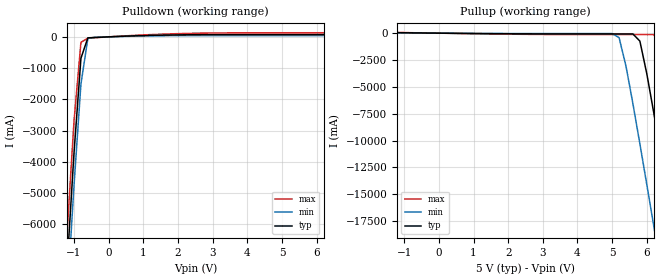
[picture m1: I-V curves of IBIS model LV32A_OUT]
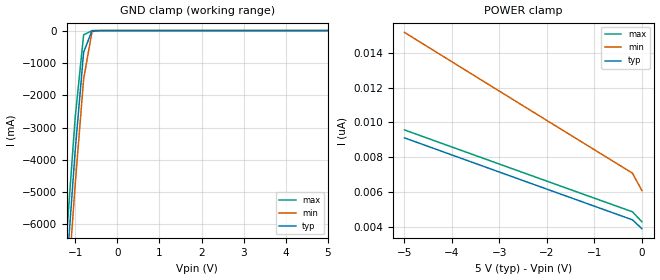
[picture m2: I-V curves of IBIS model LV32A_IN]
|   TEXAS INSTRUMENTS INCORPORATED
|   Advanced Bus Interface Group
|   IBIS Model of LV32A (Vcc=5V)
|   CMOS Quadruple 2-Input Positive-OR Gate
|   SOIC 14-pin (D) Package
[IBIS Ver]   1.1
[File Name]   lv32a_5.ibs
[File Rev]   2.0
[Date]   9/6/97
[Source]   File originated at Texas Instruments, Inc.
[Notes]   The following is an IBIS list for the LV32A.
|   - All test data contained in this file are derived from
|   hspice(tm) simulations.
|   - File created by Teruo Ishii, SLL Applications.
[Disclaimer] Property of Texas Instruments Incorporated.  Unauthorized
   reproduction and/or distribution is strictly prohibited.
   This product is protected under copyright law.
   Created 1997, (C) Copyright 1997, Texas Instruments Inc.,
   All Rights Reserved
   UNLESS THERE IS A SIGNED, WRITTEN AGREEMENT TO THE
   CONTRARY, TEXAS INSTRUMENTS ("TI") IS PROVIDING THE IBIS
   MODELS "AS IS" AND WITHOUT ANY WARRANTY, EXPRESSED OR
   IMPLIED.  TI assumes no liability for:
   1) the accuracy of the IBIS models provided to your
   company;
   2) the proper functioning of these IBIS models in your
   design or for any resulting applications; or
   3) infringement of patents, copyrights or intellectual
   property rights resulting from your use of these IBIS
   models.
   TI provides IBIS Models as a service to our customers.
   You and your company shall not distribute, sell or give
   these models to anyone else without prior written
   permission from TI.
   TI reserves the right to make changes to our products or
   to discontinue any semiconductor product or service
   without notice, and advises our customers to obtain the
   latest version of relevant information to verify, before
   placing orders, that the information being relied on is
   current.
   Please be aware that your receipt and use of the IBIS
   information provided shall serve as acceptance of these
   terms and conditions.  If you do not accept these terms,
   you should return or destroy the IBIS models and any
   other accompanying information immediately.
[Component]   LV32A(Positive-OR Gate)
[Manufacturer]  Texas Instruments
[Package]
|   typ   min   max
R_pkg   0.020   0.018   0.021
L_pkg   3.17nH   2.22nH   4.32nH
C_pkg   0.35pF   0.20pF   0.50pF
[Pin]   signal_name   model_name   R_pin   L_pin   C_pin
1   1A   LV32A_IN   0.018   4.30nH   0.50pF
2   1B   LV32A_IN   0.021   3.39nH   0.43pF
3   1Y   LV32A_OUT   0.019   2.24nH   0.26pF
4   2A   LV32A_IN   0.020   2.27nH   0.21pF
5   2B   LV32A_IN   0.020   2.22nH   0.20pF
6   2Y   LV32A_OUT   0.021   3.43nH   0.38pF
7   GND   GND   0.020   4.32nH   0.50pF
8   3Y   LV32A_OUT   0.020   4.32nH   0.50pF
9   3A   LV32A_IN   0.021   3.43nH   0.38pF
10   3B   LV32A_IN   0.020   2.22nH   0.20pF
11   4Y   LV32A_OUT   0.020   2.27nH   0.21pF
12   4A   LV32A_IN   0.019   2.24nH   0.26pF
13   4B   LV32A_IN   0.021   3.39nH   0.43pF
14   VCC   POWER   0.018   4.30nH   0.50pF
| Models and submodels in the file (2): LV32A_OUT (Output), LV32A_IN (Input)
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|   Model LV32A_OUT
[Model]   LV32A_OUT
Model_type   Output
Polarity   Non-Inverting
|variable   typ   min   max
C_comp   4.0pF   NA   NA
[Voltage range]   5.0   4.5   5.5
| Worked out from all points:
|   slope of the pulldown table from 0 to 0.75 V, typ, clamps not added: 23.2 ohm
|   slope of the pullup table from 0 to 0.75 V, typ, clamps not added: 29.8 ohm
[Pulldown]
|   Voltage   I(typ)   I(min)   I(max)
-5V       -81.99A    -82.92A    -81.08A
-1.2V     -7.334A    -8.394A    -6.29A
-1V       -3.716A    -4.76A     -2.696A
-800mV    -684.6mA   -1.507A    -174.2mA
-600mV    -32.04mA   -49.56mA   -44.95mA
-400mV    -20.26mA   -14.47mA   -29.3mA
400mV     18.84mA    13.27mA    27.19mA
2.4V      67.49mA    39.34mA    113mA
6.8V      78.69mA    44.99mA    135.4mA
10V       118mA      69.49mA    191.8mA
[Pullup]   | Note: Vtable = Vcc - Voutput
|   Voltage   I(typ)   I(min)   I(max)
-5V       63.18mA    37.18mA    178.6mA
5V        -72.29mA   -39.76mA   -130.3mA
5.2V      -72.34mA   -419.6mA   -130.3mA
5.4V      -72.63mA   -3.083A    -130.4mA
5.6V      -75.88mA   -6.59A     -130.4mA
5.8V      -740.7mA   -10.3A     -130.8mA
6.2V      -7.404A    -17.94A    -139.2mA
6.4V      -11.17A    -21.82A    -1.238A
6.8V      -18.88A    -29.62A    -8.294A
7.2V      -26.69A    -37.47A    -15.98A
7.4V      -30.61A    -41.4A     -19.88A
10V       -82.06A    -92.89A    -71.28A
[Ramp]
|Variable   typ   min   max
dV/dt_r   1.7468E+00/1.4220E-09  1.1029E+00/2.3636E-09  2.3227E+00/7.4065E-10
dV/dt_f   1.8621E+00/1.6013E-09  1.1972E+00/2.4256E-09  2.4573E+00/1.0037E-09
|   Model LV32A_IN
[Model]   LV32A_IN
Model_type   Input
Polarity   Non-Inverting
Vinl = 1.5V
Vinh = 3.5V
|variable   typ   min   max
C_comp   3.3pF   NA   NA
[Voltage Range]   5.0   4.5   5.5
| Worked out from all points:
|   GND clamp passes 1 mA (typ) near -0.46 V on its own axis
[GND_Clamp]
|   Voltage   I(typ)   I(min)   I(max)
-5V       -82A       -82.93A    -81.1A
-1.2V     -7.333A    -8.394A    -6.288A
-1V       -3.712A    -4.759A    -2.688A
-800mV    -668.4mA   -1.501A    -130.8mA
-600mV    -3.037mA   -30.13mA   -3.193mA
-400mV    -173.2uA   -104.7uA   -839.2uA
5V        3.916nA    7.599nA    3.537nA
[POWER_Clamp]   | Note: Vtable = Vcc - Voutput
|   Voltage   I(typ)   I(min)   I(max)
-5V       9.116nA    15.16nA    9.57nA
-2.4V     6.569nA    10.78nA    7.027nA
-200mV    4.423nA    7.098nA    4.883nA
0V        3.916nA    6.098nA    4.314nA
